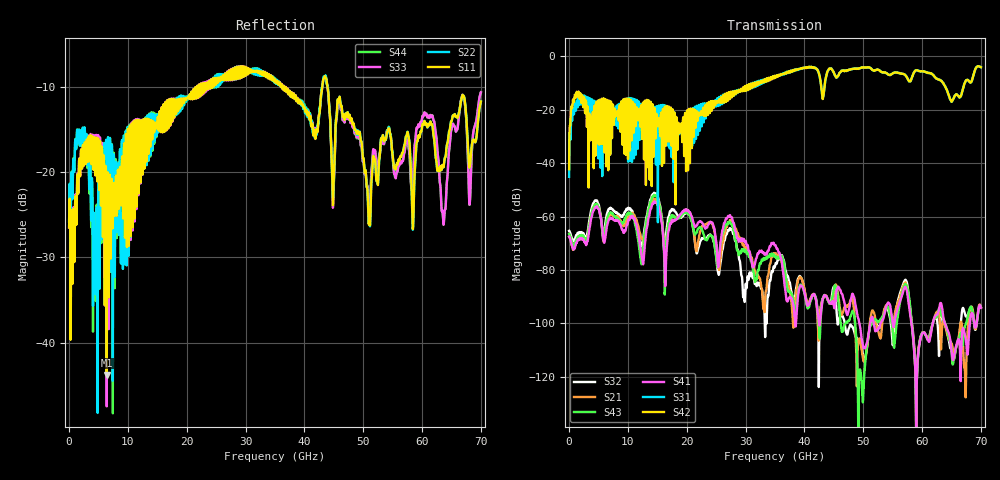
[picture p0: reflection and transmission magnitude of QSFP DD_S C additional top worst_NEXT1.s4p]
! AWR Design Environment (8415) Thu Dec 20 17:14:44 2018
! Document = 'CHANNEL TEST'
! nPorts: 4, nXvals: 7001
# HZ S DB R 50
!Freq DBS11 AngS11 DBS12 AngS12 DBS13 AngS13 DBS14 AngS14
!	DBS21 AngS21 DBS22 AngS22 DBS23 AngS23 DBS24 AngS24
!	DBS31 AngS31 DBS32 AngS32 DBS33 AngS33 DBS34 AngS34
!	DBS41 AngS41 DBS42 AngS42 DBS43 AngS43 DBS44 AngS44
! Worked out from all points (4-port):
!   7000 points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, 10 MHz to 70 GHz, reference 50 ohm
!   strongest paths, dB at 10 MHz, 17.51 GHz, 35.01 GHz, 52.51 GHz, 70 GHz:
!     S42: -42.3, -23.4, -7.5, -5.0, -4.0
!     S31: -45.1, -23.1, -7.6, -5.0, -4.0
!     S41: -67.4, -61.4, -70.7, -101.9, -94.2
!     S43: -66.5, -59.4, -75.0, -99.3, -93.9
!     S21: -67.5, -59.7, -74.0, -102.7, -94.0
!     S32: -65.3, -57.1, -78.5, -101.0, -93.8
!   lowest |S11| = -43.8 dB at 6.41 GHz (marker M1), VSWR 1.01, Z = 50.5 - j0.428 ohm
!   |S11| at or under -10 dB: start of sweep to 21.78 GHz; 36.52 GHz to 43.04 GHz (6.515 GHz wide, 16.4 % of centre); 43.91 GHz to end of sweep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
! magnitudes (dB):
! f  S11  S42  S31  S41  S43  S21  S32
! 10 MHz  -26.5  -42.3  -45.1  -67.4  -66.5  -67.5  -65.3
! 1.29 GHz  -24.2  -13.3  -16.8  -69.8  -68.6  -69.0  -66.9
! 6.41 GHz  -43.8  -21.7  -18.7  -63.8  -61.0  -62.0  -59.1
! 12.28 GHz  -14.2  -18.7  -23.0  -74.3  -77.8  -68.2  -71.1
! 14.65 GHz  -14.3  -27.2  -19.9  -54.7  -52.3  -53.7  -51.4
! 25.45 GHz  -9.0  -17.1  -16.1  -77.5  -75.5  -79.9  -81.7
! 70 GHz  -11.8  -4.0  -4.0  -94.2  -93.9  -94.0  -93.8
